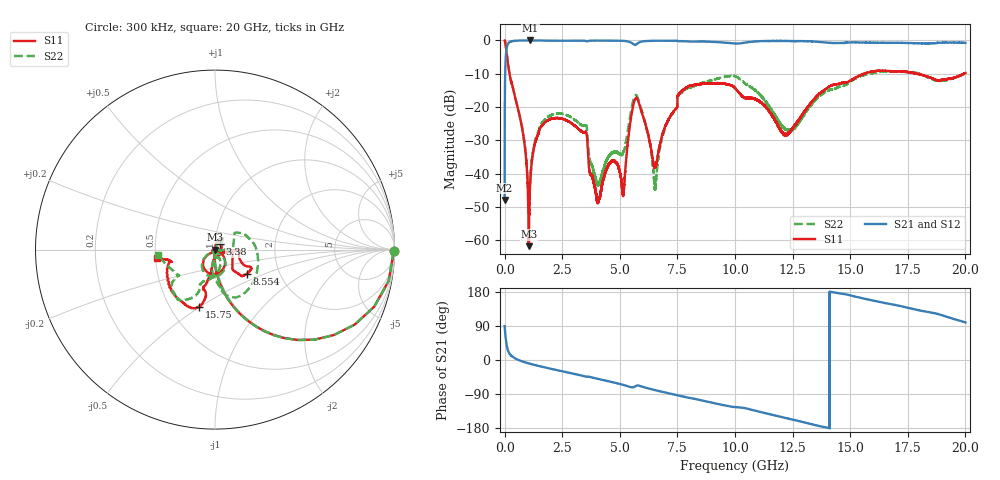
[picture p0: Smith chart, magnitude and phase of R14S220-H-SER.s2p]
!{R14S220}
!Johanson Technology Inc.
!www.johansontechnology.com
!Test Board Conditions:
!Substrate Type  RO4350B
!Substrate Thickness  20 mil
!Substrate Dk  3.66
!TL Type: GCPW
!TL Trace Width  36 mil
!TL Gap  12 mil
!Electrode orientation  Horizontal
!DUT TOPOLOGY	SERIES
!Mounting Pad LxW  26x36 mil
! Created Wed Nov 25 17:33:21 2020
! 2 Port Network Data from SP1.SP block
! freq  magS11  angS11  magS21  angS21  magS12  angS12  magS22  angS22
# khz S ma R 50
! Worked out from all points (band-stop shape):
!   20001 points, 300 kHz to 20 GHz, reference 50 ohm
!   highest |S21| = 0.00 dB at 1.109 GHz (marker M1); lowest = -47.9 dB at 300 kHz (marker M2)
!   |S21| within 3 dB of the highest: 74.5 MHz to end of sweep
!   lowest |S11| = -61.8 dB at 1.053 GHz (marker M3), VSWR 1.00, Z = 49.9 + j0.0119 ohm
!   |S11| at or under -10 dB: 213.7 MHz to 15.59 GHz (15.38 GHz wide, 195 % of centre); 15.5994 GHz to 15.60434 GHz (4.936 MHz wide, 0.0316 % of centre); 17.87 GHz to 19.93 GHz (2.058 GHz wide, 10.9 % of centre)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
!   |S22| runs from -51.5 to 0.0 dB; largest |S21 - S12| = 0.02
!   S11 on the Smith chart (normalised r, x): 300 kHz: open; 3.38 GHz: 1.05, +0.07; 8.554 GHz: 1.36, -0.39; 15.75 GHz: 0.70, -0.50; 20 GHz: 0.51, -0.05
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300  0.9968 -0.4  0.004041 89.5  0.004134 89.0  0.9957 -0.5
146300  0.4442 -64.7  0.8924 25.2  0.8933 25.1  0.4472 -64.6
787300  0.04274 -94.3  0.9981 -4.1  0.9979 -4.1  0.04405 -91.8
1053300  0.0008167 171.6  0.9984 -9.1  0.9993 -9.1  0.002929 -9.3
1109300  0.007062 92.2  0.9997 -10.0  0.9987 -10.0  0.007284 58.3
1665300  0.05459 71.1  0.9957 -18.4  0.9951 -18.4  0.06024 70.6
3334300  0.04299 50.9  0.9929 -41.0  0.9936 -40.9  0.05368 43.6
3380300  0.04222 49.2  0.9931 -41.6  0.9933 -41.6  0.05248 41.5
4059300  0.003885 118.6  0.9953 -49.9  0.9955 -49.9  0.006761 -44.2
4667300  0.01518 -162.4  0.9939 -58.3  0.9941 -58.3  0.02051 -116.6
5151300  0.004982 -90.9  0.9858 -65.7  0.9864 -65.8  0.02111 -74.9
5689300  0.1355 -90.0  0.8647 -68.9  0.8638 -68.8  0.1519 -93.5
6502300  0.01282 -91.9  0.9891 -79.1  0.9899 -79.1  0.007073 -105.5
6667300  0.02064 -28.6  0.9901 -81.5  0.9904 -81.5  0.01665 -5.1
7600300  0.1627 -48.0  0.9784 -94.4  0.9787 -94.3  0.1575 36.5
8554300  0.2228 -37.7  0.964 -106.6  0.9636 -106.6  0.2297 1.4
1.00003e7  0.193 -28.0  0.8997 -124.3  0.8978 -124.3  0.2913 -66.0
1.21903e7  0.03948 -53.8  0.9816 -152.9  0.984 -152.8  0.04659 -84.2
1.33343e7  0.1192 -100.1  0.9679 -169.6  0.9697 -169.6  0.1098 -76.8
1.57543e7  0.3296 -105.3  0.9257 159.8  0.9314 160.0  0.3129 -118.1
1.66673e7  0.3457 -118.7  0.9214 148.5  0.9117 148.3  0.3475 -126.7
2e7  0.325 -171.6  0.9186 99.1  0.9186 99.6  0.3221 -174.5
